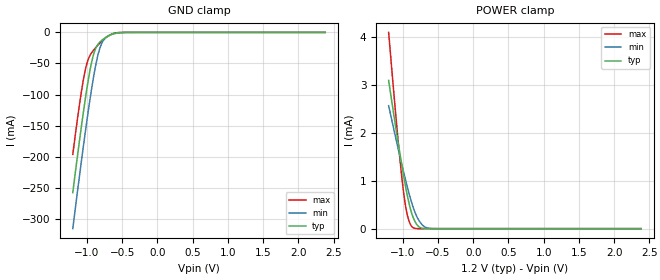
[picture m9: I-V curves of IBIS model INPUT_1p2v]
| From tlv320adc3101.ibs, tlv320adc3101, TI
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|   INPUT_1p2v
[Model]   INPUT_1p2v
Model_type   Input
Vinl = 0.36
Vinh = 0.84
|   typ   min   max
C_comp   1.022pF   1.010pF   1.056pF
[Voltage Range]   1.2   1.1   1.3
[Temperature Range]   27   85   -40
[Power Clamp Reference]   1.2   1.1   1.3
[GND Clamp Reference]   -0   -0   -0
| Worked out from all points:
|   GND clamp passes 1 mA (typ) near -0.58 V on its own axis
|   POWER clamp passes 1 mA (typ) near -0.97 V on its own axis
[GND Clamp]
|   Voltage   I(typ)   I(min)   I(max)
-1.2V     -257.8mA   -315.8mA   -196.3mA
-1.11V    -178.6mA   -235.4mA   -120.2mA
-1.038V   -119.2mA   -173.6mA   -69.12mA
-984mV    -79.23mA   -129.6mA   -44.34mA
-930mV    -46.66mA   -88.84mA   -32.31mA
-876mV    -26.07mA   -53.68mA   -24.64mA
-822mV    -16.32mA   -27.71mA   -17.99mA
-768mV    -10.92mA   -13.34mA   -12.06mA
-714mV    -6.903mA   -6.996mA   -7.064mA
-624mV    -2.307mA   -2.419mA   -1.729mA
-534mV    -409.5uA   -566.6uA   -175.5uA
2.382V    0A         0A         0A
[POWER Clamp]
|   Voltage   I(typ)   I(min)   I(max)
-1.2V     3.094mA    2.568mA    4.098mA
-1.074V   1.877mA    1.728mA    1.973mA
-1.02V    1.385mA    1.382mA    1.165mA
-984mV    1.075mA    1.159mA    711uA
-930mV    656.3uA    841uA      253.6uA
-894mV    428.5uA    645.9uA    94.27uA
-858mV    256uA      471.3uA    24.6uA
-804mV    92.62uA    263.6uA    2.247uA
-750mV    21.06uA    125.8uA    182.4nA
-678mV    1.797uA    29.97uA    1.807nA
-606mV    132.4nA    4.222uA    0A
2.382V    0A         0A         0A
